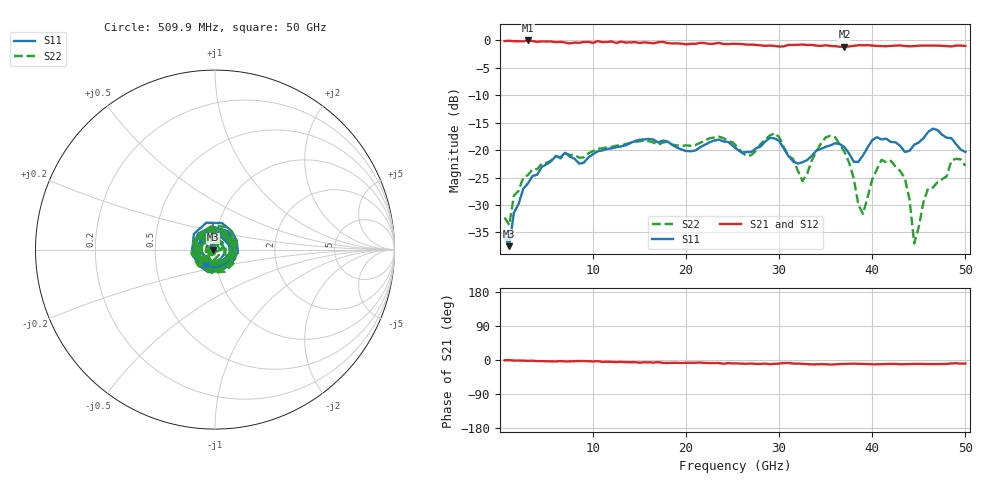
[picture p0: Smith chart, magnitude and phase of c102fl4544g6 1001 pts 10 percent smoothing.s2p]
! 8/14/2019 7:28:27 AM
! Y:\TERRY-ANALYZER-FILES\CONICAL DATA FOR CLAUDE\C102FL4544G6 1001 PTS 10 PERCENT SMOOTHING.S2P
! CHANNEL.1
! TR.MEASUREMENT
! CORRECTED.DATA
# GHZ S RI R 50.0
! FREQ.GHZ  S11RE  S11IM  S21RE  S21IM  S12RE  S12IM  S22RE  S22IM
!; PortSelection: Port_12
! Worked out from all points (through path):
!   100 points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, 509.9 MHz to 50 GHz, reference 50 ohm
!   highest |S21| = 0.00 dB at 3.009 GHz (marker M1); lowest = -1.1 dB at 37 GHz (marker M2)
!   group delay of S21, straight-line fit = 550 fs
!   lowest |S11| = -37.5 dB at 1.01 GHz (marker M3), VSWR 1.03, Z = 48.7 - j0.0232 ohm
!   |S11| at or under -10 dB: start of sweep to end of sweep
!   |S22| runs from -37.0 to -16.9 dB; largest |S21 - S12| = 0.027
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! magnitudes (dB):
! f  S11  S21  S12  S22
! 509.9 MHz  -35.6  -0.1  -0.1  -32.3
! 1.01 GHz  -37.5  -0.1  -0.1  -33.7
! 1.51 GHz  -31.4  -0.1  -0.1  -28.3
! 3.009 GHz  -26.1  0.0  0.0  -24.5
! 6.009 GHz  -21.1  -0.3  -0.3  -21.0
! 9.008 GHz  -22.3  -0.3  -0.3  -21.3
! 17.51 GHz  -18.2  -0.2  -0.4  -18.6
! 25.5 GHz  -19.9  -0.6  -0.7  -19.4
! 27 GHz  -20.3  -0.7  -0.7  -20.9
! 29.5 GHz  -17.8  -1.0  -1.1  -16.9
! 32.5 GHz  -22.2  -0.7  -0.8  -25.6
! 33.5 GHz  -21.0  -0.8  -0.8  -21.9
! 35.5 GHz  -19.1  -1.0  -0.9  -17.4
! 37 GHz  -19.4  -1.1  -1.1  -20.3
! 39 GHz  -20.9  -0.9  -0.9  -31.6
! 41 GHz  -18.0  -1.0  -1.0  -21.8
! 42 GHz  -18.5  -1.0  -1.0  -21.9
! 43.5 GHz  -20.3  -1.0  -1.1  -25.2
! 44.5 GHz  -19.0  -1.0  -1.1  -37.0
! 46 GHz  -16.7  -0.9  -0.9  -27.0
! 48.5 GHz  -17.8  -1.1  -1.0  -21.9
! 50 GHz  -20.3  -1.0  -1.0  -22.8
